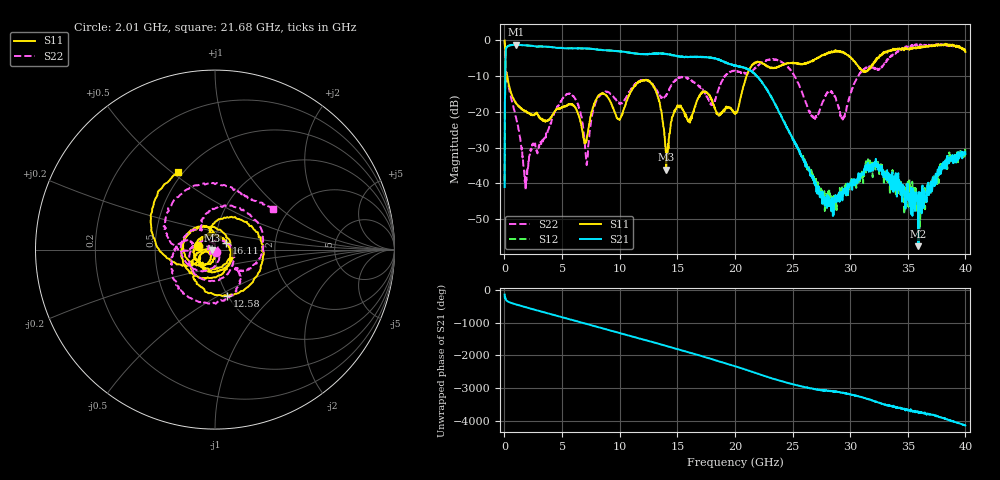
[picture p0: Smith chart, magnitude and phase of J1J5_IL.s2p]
!Agilent Technologies,N5230A,US43500312,A.07.50.67
!Agilent N5230A: A.07.50.67
!Date: Thursday, March 05, 2015 11:30:20
!Correction: S11(Full 2 Port(1,2))
!S21(Full 2 Port(1,2))
!S12(Full 2 Port(1,2))
!S22(Full 2 Port(1,2))
!S2P File: Measurements: S11, S21, S12, S22:
# Hz S  dB  R 50
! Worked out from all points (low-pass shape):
!   1601 points, 10 MHz to 40 GHz, reference 50 ohm
!   highest |S21| = -1.29 dB at 984.8 MHz (marker M1); lowest = -57.5 dB at 35.93 GHz (marker M2)
!   |S21| within 3 dB of the highest: 90.88 MHz to 14.72 GHz (14.63 GHz wide, 198 % of centre); 14.75727 GHz to 14.81189 GHz (54.62 MHz wide, 0.369 % of centre)
!   lowest |S11| = -36.2 dB at 14.03 GHz (marker M3), VSWR 1.03, Z = 48.5 - j0.408 ohm
!   |S11| at or under -10 dB: 81.43 MHz to 123.3 MHz (41.9 MHz wide, 40.9 % of centre); 234.9 MHz to 21.01 GHz (20.78 GHz wide, 196 % of centre)
!   |S22| runs from -41.9 to -0.1 dB; largest |S21 - S12| = 0.013
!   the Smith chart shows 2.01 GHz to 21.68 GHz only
!   S11 on the Smith chart (normalised r, x): 2.01 GHz: 0.83, +0.03; 12.58 GHz: 0.99, -0.55; 16.11 GHz: 1.13, +0.08; 21.68 GHz: 0.47, +0.53
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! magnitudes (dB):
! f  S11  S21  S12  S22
! 10 MHz  -0.1  -41.0  -39.4  -0.1
! 284.9 MHz  -10.9  -1.7  -1.7  -11.4
! 984.8 MHz  -17.4  -1.3  -1.3  -21.4
! 2.01 GHz  -20.3  -1.5  -1.5  -35.8
! 5.234 GHz  -18.5  -2.3  -2.2  -15.6
! 6.683 GHz  -24.1  -2.3  -2.3  -21.4
! 7.158 GHz  -27.1  -2.3  -2.3  -34.3
! 8.283 GHz  -15.1  -2.7  -2.7  -15.5
! 9.933 GHz  -22.2  -3.1  -3.1  -17.5
! 12.58 GHz  -11.6  -3.8  -3.8  -11.3
! 13.36 GHz  -16.3  -3.6  -3.7  -14.8
! 14.03 GHz  -36.2  -3.9  -3.8  -15.5
! 16.11 GHz  -23.0  -4.7  -4.6  -10.9
! 18.01 GHz  -16.5  -4.9  -4.9  -18.2
! 20 GHz  -20.2  -7.1  -7.2  -8.5
! 21.68 GHz  -6.4  -9.3  -9.3  -8.0
! 24.35 GHz  -6.6  -23.3  -23.5  -6.8
! 26.68 GHz  -5.8  -38.2  -37.3  -21.1
! 28.63 GHz  -3.2  -43.9  -47.2  -15.6
! 33.35 GHz  -2.9  -38.3  -38.0  -5.1
! 35.93 GHz  -2.2  -57.5  -44.2  -1.5
! 40 GHz  -3.3  -31.8  -31.3  -2.4
